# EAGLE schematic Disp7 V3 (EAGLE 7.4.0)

## Sheet 1 of 5: Powersupply
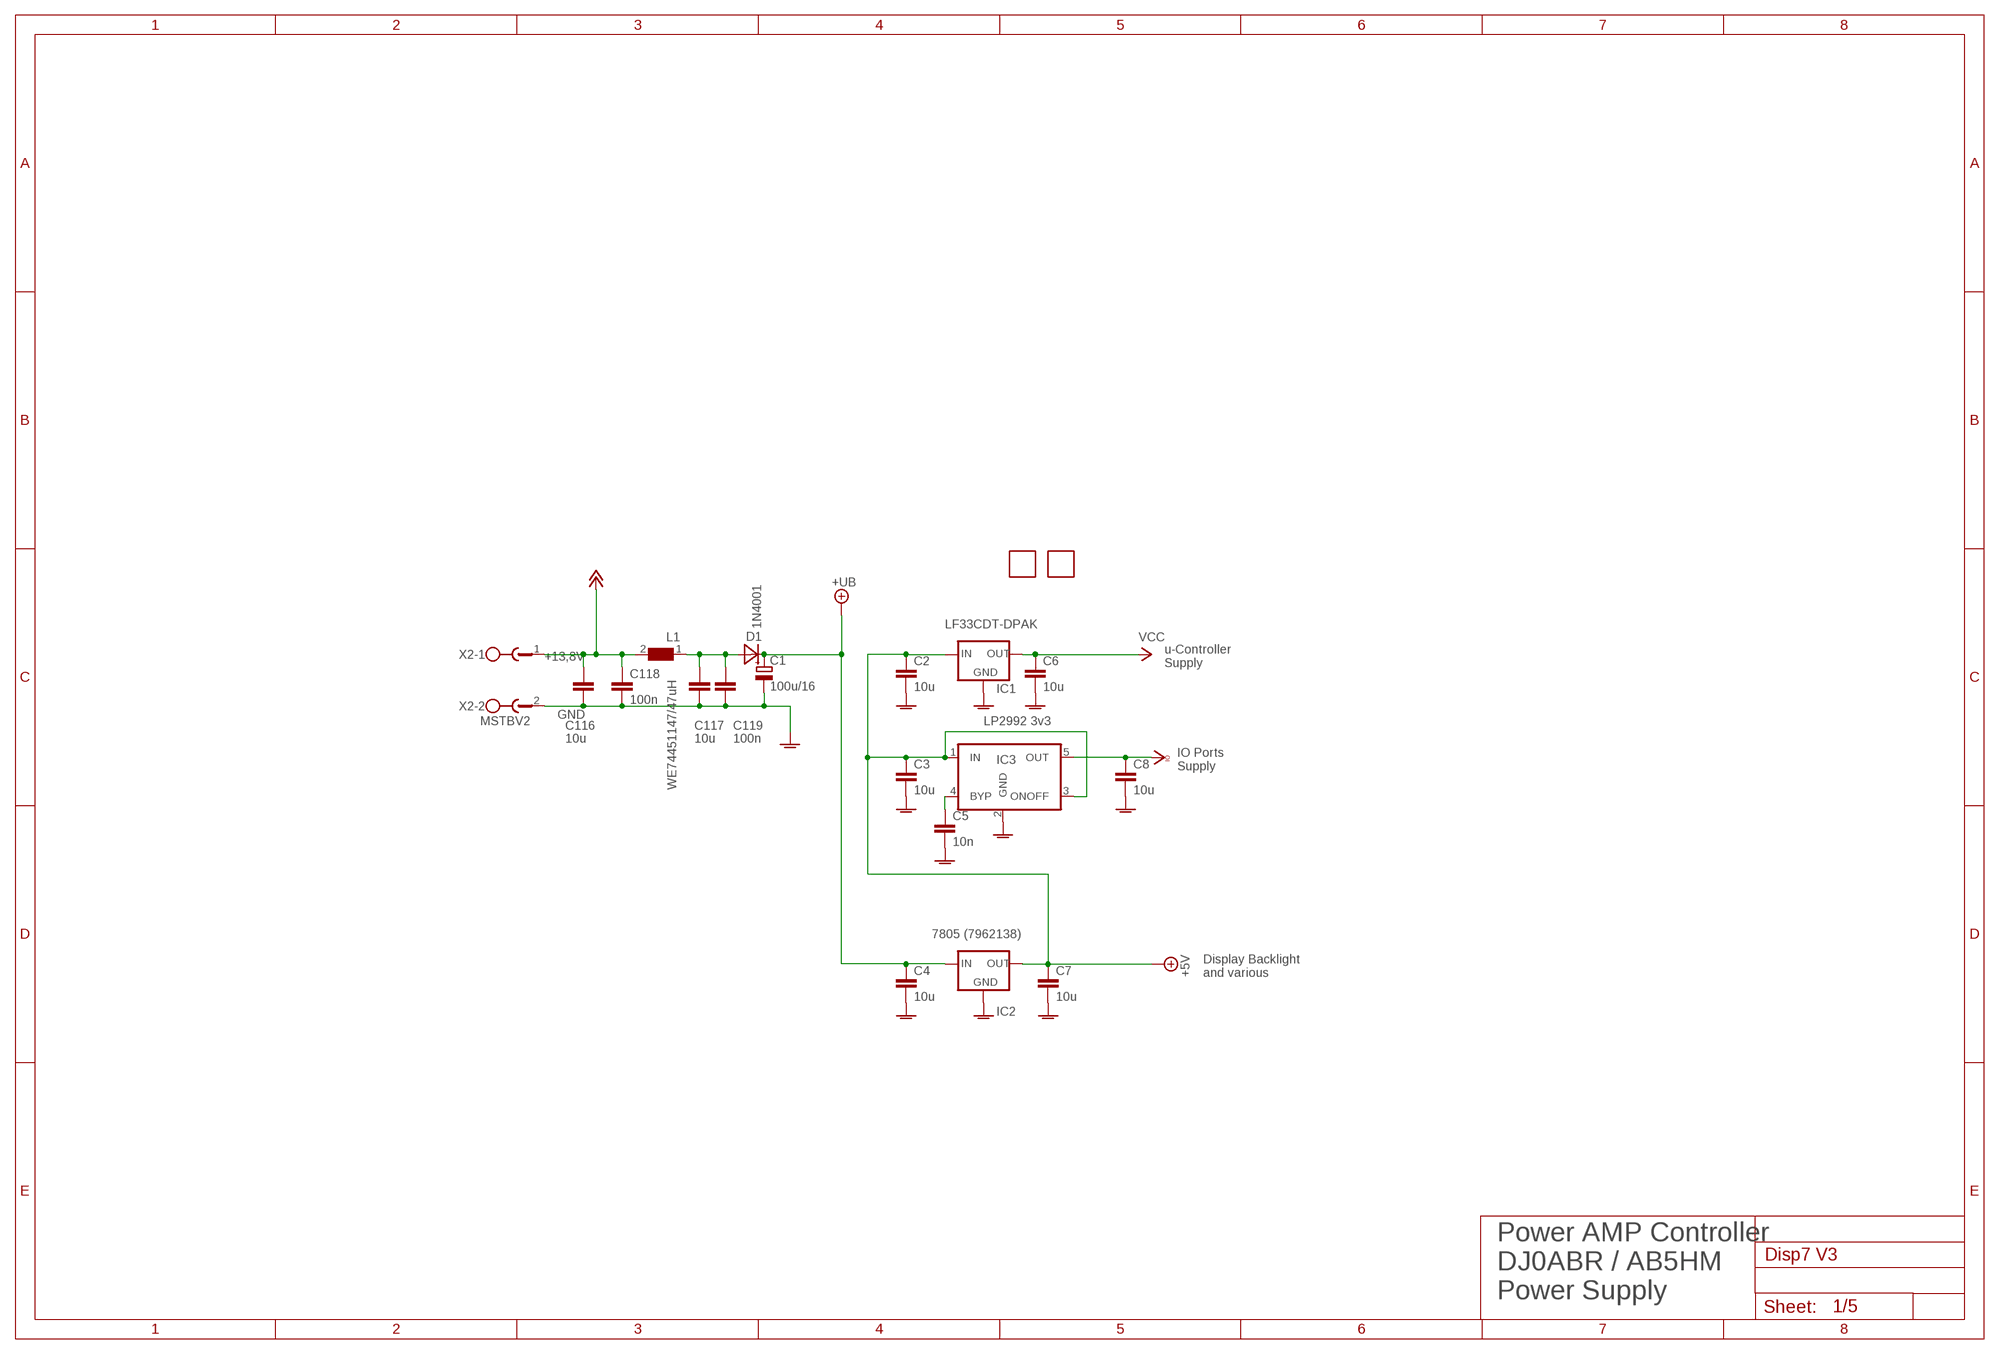
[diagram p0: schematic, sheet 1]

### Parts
C1  100u/16  CPOL-EUE2.5-7  [E2,5-7]
C2  10u  C-EUC0805  [C0805]
C3  10u  C-EUC0805  [C0805]
C4  10u  C-EUC0805  [C0805]
C5  10n  C-EUC0805  [C0805]
C6  10u  C-EUC0603  [C0603]
C7  10u  C-EUC0603  [C0603]
C8  10u  C-EUC0603  [C0603]
C116  10u  C-EUC0805  [C0805]
C117  10u  C-EUC0805  [C0805]
C118  100n  C-EUC0805  [C0805]
C119  100n  C-EUC0805  [C0805]
D1  1N4001  DIODE_GROSSSMD  [MELF]
FID1  FIDUCIAL  [FIDUCIAL]
FID2  FIDUCIAL  [FIDUCIAL]
IC1  LF33CDT-DPAK  LP2950CDT-5.0  [DPACK]
IC2  7805 (7962138)  78XXSWITCHREG  [78SR_SWITCHREG]
IC3  LP2992 3v3  UREG5  [SOT23-5]
L1  WE74451147/47uH  WE-PD3-74451147_S  [S]
X2  MSTBV2  [MSTBV2]

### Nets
+5V: C2.1 C3.1 C7.1 IC1.1(IN) IC2.3(OUT) IC3.1(IN) IC3.3(ONOFF) ; also sheet 3,4
+UB [Supply]: C1.+ C4.1 D1.1(C) IC2.1(IN) ; also sheet 3
AGND [AGND]: C1.- C2.2 C3.2 C4.2 C5.2 C6.2 C7.2 C8.2 C116.2 C117.2 C118.2 C119.2 IC1.4(GND) IC2.2(GND) IC3.2(GND) X2.2 ; supply symbol labelled  ; also sheet 2,3,4,5
N$47 [Supply]: C117.1 C119.1 D1.2(A) L1.1
N$125: C5.1 IC3.4(BYP)
PLUSZWOELF [Supply]: C116.1 C118.1 L1.2 X2.1 ; supply symbol labelled +12V ; also sheet 2
VCC [Supply]: C6.1 IC1.3(OUT) ; also sheet 2,4,5
VCCIO [Supply]: C8.1 IC3.5(OUT) ; supply symbol labelled  ; also sheet 3,4
Unconnected: FID1.P$1 FID2.P$1

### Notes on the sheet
- +13,8V
- u-Controller 
  Supply
- GND
- IO Ports
  Supply
- Display Backlight
  and various
- Power AMP Controller
  DJ0ABR / AB5HM
  Power Supply

## Sheet 2 of 5: IO Ports LED,PTT,Switch
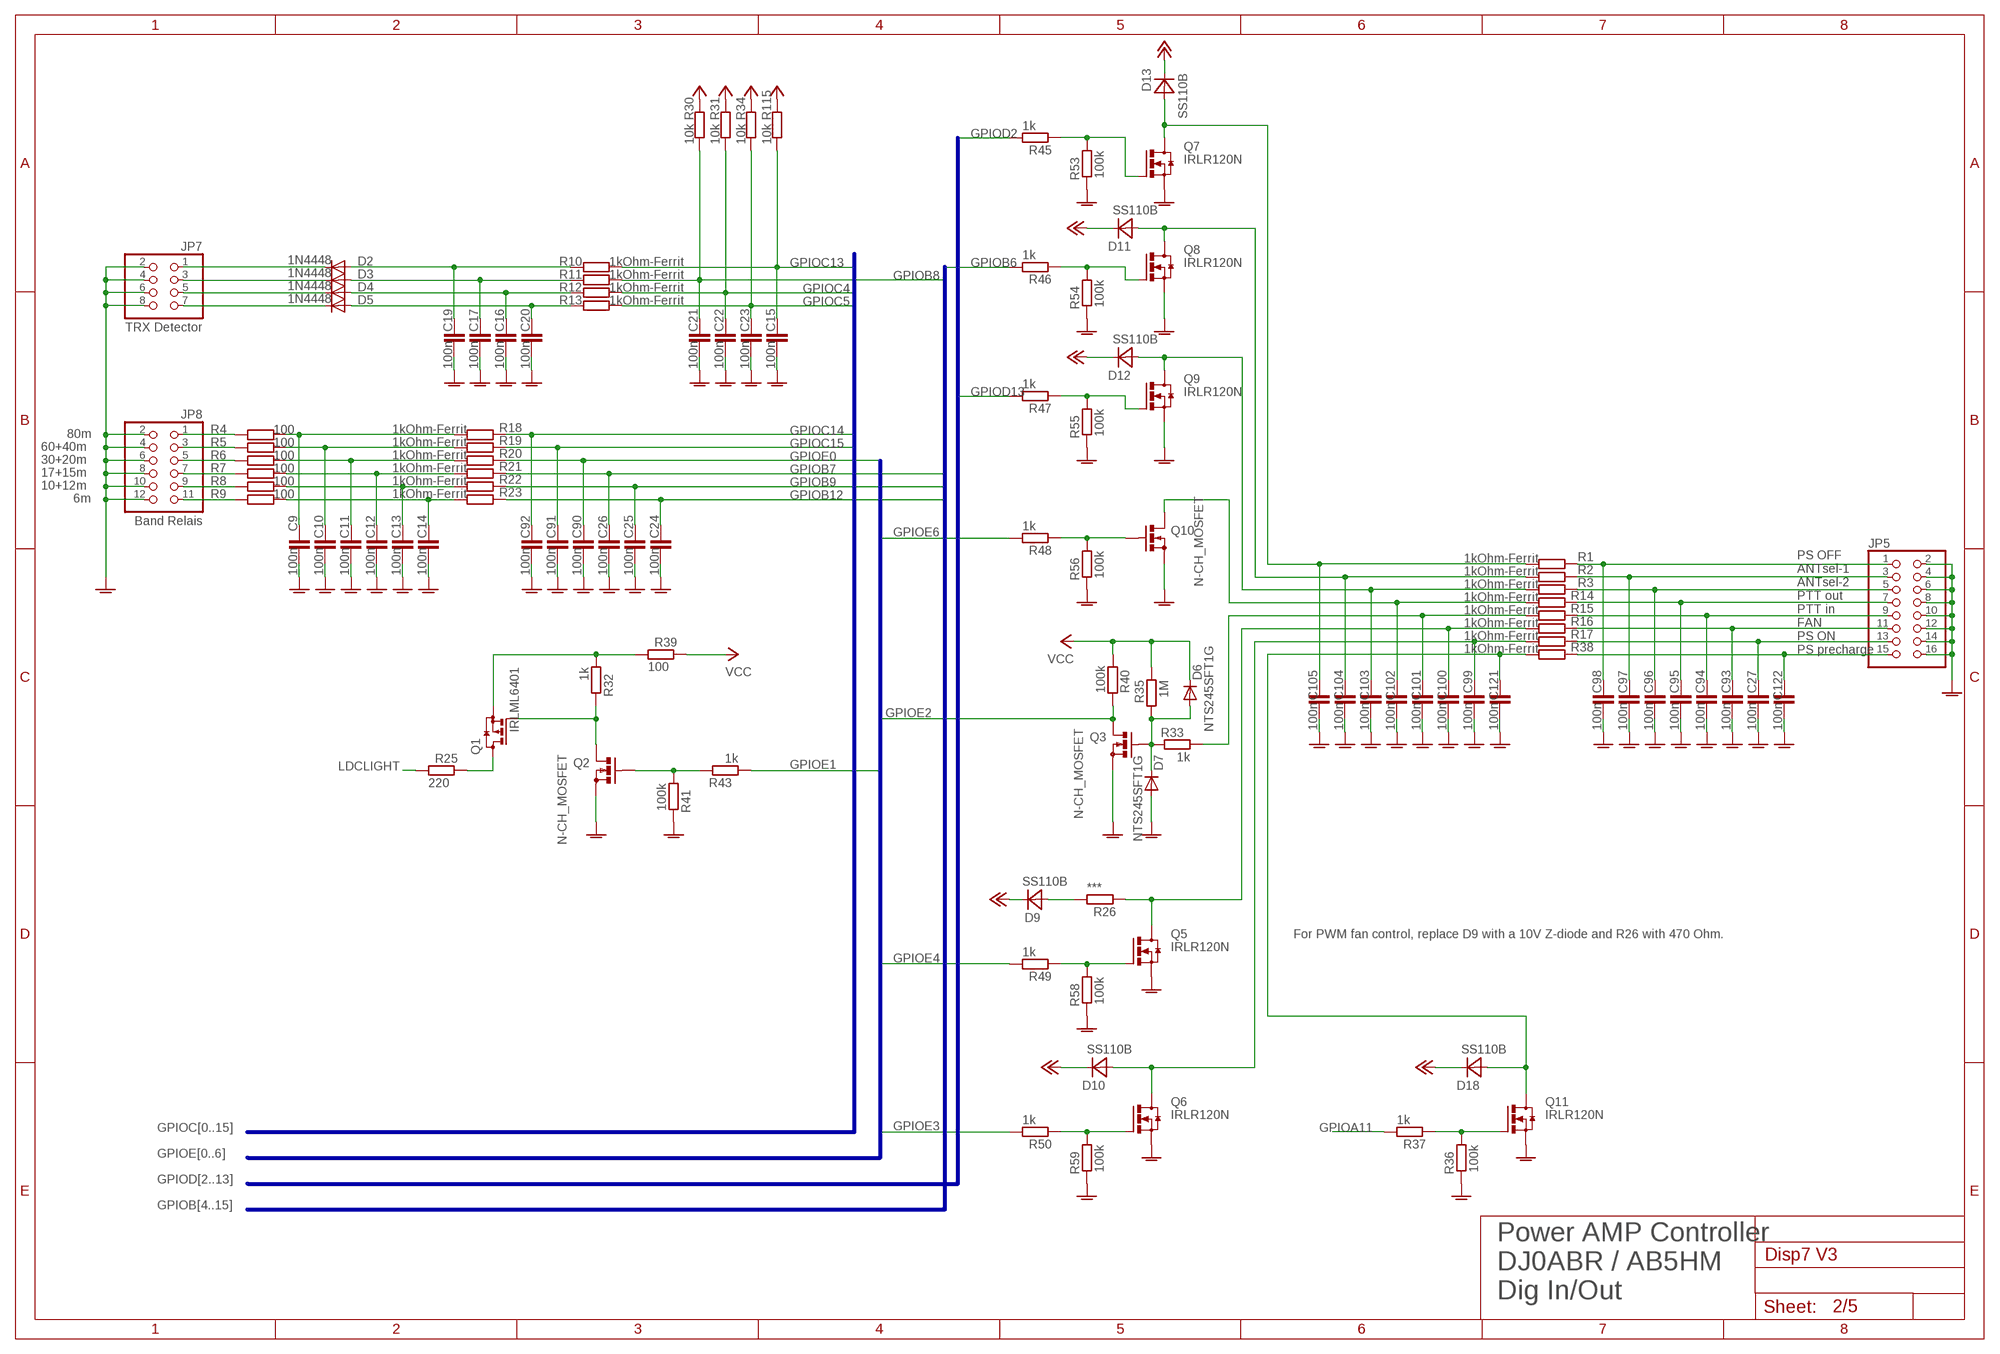
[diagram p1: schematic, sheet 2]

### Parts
C9  100n  C-EUC0805  [C0805]
C10  100n  C-EUC0805  [C0805]
C11  100n  C-EUC0805  [C0805]
C12  100n  C-EUC0805  [C0805]
C13  100n  C-EUC0805  [C0805]
C14  100n  C-EUC0805  [C0805]
C15  100n  C-EUC0805  [C0805]
C16  100n  C-EUC0805  [C0805]
C17  100n  C-EUC0805  [C0805]
C19  100n  C-EUC0805  [C0805]
C20  100n  C-EUC0805  [C0805]
C21  100n  C-EUC0805  [C0805]
C22  100n  C-EUC0805  [C0805]
C23  100n  C-EUC0805  [C0805]
C24  100n  C-EUC0805  [C0805]
C25  100n  C-EUC0805  [C0805]
C26  100n  C-EUC0805  [C0805]
C27  100n  C-EUC0805  [C0805]
C90  100n  C-EUC0805  [C0805]
C91  100n  C-EUC0805  [C0805]
C92  100n  C-EUC0805  [C0805]
C93  100n  C-EUC0805  [C0805]
C94  100n  C-EUC0805  [C0805]
C95  100n  C-EUC0805  [C0805]
C96  100n  C-EUC0805  [C0805]
C97  100n  C-EUC0805  [C0805]
C98  100n  C-EUC0805  [C0805]
C99  100n  C-EUC0805  [C0805]
C100  100n  C-EUC0805  [C0805]
C101  100n  C-EUC0805  [C0805]
C102  100n  C-EUC0805  [C0805]
C103  100n  C-EUC0805  [C0805]
C104  100n  C-EUC0805  [C0805]
C105  100n  C-EUC0805  [C0805]
C121  100n  C-EUC0805  [C0805]
C122  100n  C-EUC0805  [C0805]
D2  1N4448  DIODE-MINIMELF  [MINIMELF]
D3  1N4448  DIODE-MINIMELF  [MINIMELF]
D4  1N4448  DIODE-MINIMELF  [MINIMELF]
D5  1N4448  DIODE-MINIMELF  [MINIMELF]
D6  NTS245SFT1G  DIODE-MINIMELF  [MINIMELF]
D7  NTS245SFT1G  DIODE-MINIMELF  [MINIMELF]
D9  SS110B  DIODE_GROSSSMD  [MELF]
D10  SS110B  DIODE_GROSSSMD  [MELF]
D11  SS110B  DIODE_GROSSSMD  [MELF]
D12  SS110B  DIODE_GROSSSMD  [MELF]
D13  SS110B  DIODE_GROSSSMD  [MELF]
D18  SS110B  DIODE_GROSSSMD  [MELF]
JP5  PINHD-2X8/90  [2X08/90]
JP7  TRX Detector  PINHD-2X4/90  [2X04/90]
JP8  Band Relais  PINHD-2X6/90  [2X06/90]
Q1  IRLML6401  BSS84  [SOT23]
Q2  N-CH_MOSFET  BS170_SMD  [SOT23]
Q3  N-CH_MOSFET  BS170_SMD  [SOT23]
Q5  IRLR120N  [D-PAK_TO252AA]
Q6  IRLR120N  [D-PAK_TO252AA]
Q7  IRLR120N  [D-PAK_TO252AA]
Q8  IRLR120N  [D-PAK_TO252AA]
Q9  IRLR120N  [D-PAK_TO252AA]
Q10  N-CH_MOSFET  BS170_SMD  [SOT23]
Q11  IRLR120N  [D-PAK_TO252AA]
R1  1kOhm-Ferrit  R-EU_R0805  [R0805]
R2  1kOhm-Ferrit  R-EU_R0805  [R0805]
R3  1kOhm-Ferrit  R-EU_R0805  [R0805]
R4  100  R-EU_R0805  [R0805]
R5  100  R-EU_R0805  [R0805]
R6  100  R-EU_R0805  [R0805]
R7  100  R-EU_R0805  [R0805]
R8  100  R-EU_R0805  [R0805]
R9  100  R-EU_R0805  [R0805]
R10  1kOhm-Ferrit  R-EU_R0805  [R0805]
R11  1kOhm-Ferrit  R-EU_R0805  [R0805]
R12  1kOhm-Ferrit  R-EU_R0805  [R0805]
R13  1kOhm-Ferrit  R-EU_R0805  [R0805]
R14  1kOhm-Ferrit  R-EU_R0805  [R0805]
R15  1kOhm-Ferrit  R-EU_R0805  [R0805]
R16  1kOhm-Ferrit  R-EU_R0805  [R0805]
R17  1kOhm-Ferrit  R-EU_R0805  [R0805]
R18  1kOhm-Ferrit  R-EU_R0805  [R0805]
R19  1kOhm-Ferrit  R-EU_R0805  [R0805]
R20  1kOhm-Ferrit  R-EU_R0805  [R0805]
R21  1kOhm-Ferrit  R-EU_R0805  [R0805]
R22  1kOhm-Ferrit  R-EU_R0805  [R0805]
R23  1kOhm-Ferrit  R-EU_R0805  [R0805]
R25  220  R-EU_R0805  [R0805]
R26  ***  R-EU_R0805  [R0805]
R30  10k  R-EU_R0805  [R0805]
R31  10k  R-EU_R0805  [R0805]
R32  1k  R-EU_R0805  [R0805]
R33  1k  R-EU_R0805  [R0805]
R34  10k  R-EU_R0805  [R0805]
R35  1M  R-EU_R0805  [R0805]
R36  100k  R-EU_R0805  [R0805]
R37  1k  R-EU_R0805  [R0805]
R38  1kOhm-Ferrit  R-EU_R0805  [R0805]
R39  100  R-EU_R0805  [R0805]
R40  100k  R-EU_R0805  [R0805]
R41  100k  R-EU_R0805  [R0805]
R43  1k  R-EU_R0805  [R0805]
R45  1k  R-EU_R0805  [R0805]
R46  1k  R-EU_R0805  [R0805]
R47  1k  R-EU_R0805  [R0805]
R48  1k  R-EU_R0805  [R0805]
R49  1k  R-EU_R0805  [R0805]
R50  1k  R-EU_R0805  [R0805]
R53  100k  R-EU_R0805  [R0805]
R54  100k  R-EU_R0805  [R0805]
R55  100k  R-EU_R0805  [R0805]
R56  100k  R-EU_R0805  [R0805]
R58  100k  R-EU_R0805  [R0805]
R59  100k  R-EU_R0805  [R0805]
R115  10k  R-EU_R0805  [R0805]

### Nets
AGND [AGND]: C9.2 C10.2 C11.2 C12.2 C13.2 C14.2 C15.2 C16.2 C17.2 C19.2 C20.2 C21.2 C22.2 C23.2 C24.2 C25.2 C26.2 C27.2 C90.2 C91.2 C92.2 C93.2 C94.2 C95.2 C96.2 C97.2 C98.2 C99.2 C100.2 C101.2 C102.2 C103.2 C104.2 C105.2 C121.2 C122.2 D7.A JP5.2 JP5.4 JP5.6 JP5.8 JP5.10 JP5.12 JP5.14 JP5.16 JP7.2 JP7.4 JP7.6 JP7.8 JP8.2 JP8.4 JP8.6 JP8.8 JP8.10 JP8.12 Q2.2(S) Q3.2(S) Q5.3(S) Q6.3(S) Q7.3(S) Q8.3(S) Q9.3(S) Q10.2(S) Q11.3(S) R36.2 R41.2 R53.2 R54.2 R55.2 R56.2 R58.2 R59.2 ; supply symbol labelled  ; also sheet 1,3,4,5
GPIOA11: R37.1 ; also sheet 4
GPIOB6: R46.1 ; also sheet 4
GPIOB7: C26.1 R21.1 ; also sheet 4
GPIOB8: C21.1 R11.2 R30.1 ; also sheet 4
GPIOB9: C25.1 R22.1 ; also sheet 4
GPIOB12: C24.1 R23.1 ; also sheet 4
GPIOC4: C22.1 R12.2 R31.1 ; also sheet 4
GPIOC5: C23.1 R13.2 R34.1 ; also sheet 4
GPIOC13: C15.1 R10.2 R115.1 ; also sheet 4
GPIOC14: C92.1 R18.1 ; also sheet 4
GPIOC15: C91.1 R19.1 ; also sheet 4
GPIOD2: R45.1 ; also sheet 4
GPIOD13: R47.1 ; also sheet 4
GPIOE0: C90.1 R20.1 ; also sheet 4
GPIOE1: R43.1 ; also sheet 4
GPIOE2: Q3.3(D) R40.1 ; also sheet 4
GPIOE3: R50.1 ; also sheet 4
GPIOE4: R49.1 ; also sheet 4
GPIOE6: R48.1 ; also sheet 4
LDCLIGHT: R25.1 ; also sheet 4
N$1: Q10.1(G) R48.2 R56.1
N$2: C102.1 Q10.3(D) R14.2
N$4: D6.A D7.C Q3.1(G) R33.2 R35.2
N$6: Q2.1(G) R41.1 R43.2
N$8: Q1.1(G) Q2.3(D) R32.2
N$10: Q1.3(D) R25.2
N$12: JP8.1 R4.1
N$14: C121.1 D18.2(A) Q11.4(D) R38.2
N$27: Q11.1(G) R36.1 R37.2
N$29: C122.1 JP5.15 R38.1
N$33: C98.1 JP5.1 R1.1
N$45: Q9.1(G) R47.2 R55.1
N$46: C103.1 D12.2(A) Q9.4(D) R3.2
N$50: C97.1 JP5.3 R2.1
N$51: C96.1 JP5.5 R3.1
N$52: C95.1 JP5.7 R14.1
N$56: C94.1 JP5.9 R15.1
N$57: C93.1 JP5.11 R16.1
N$58: D3.C JP7.3
N$59: D4.C JP7.5
N$60: D5.C JP7.7
N$63: C27.1 JP5.13 R17.1
N$65: D9.2(A) R26.1
N$90: C9.1 R4.2 R18.2
N$94: C14.1 R9.2 R23.2
N$95: C13.1 R8.2 R22.2
N$98: C12.1 R7.2 R21.2
N$99: C11.1 R6.2 R20.2
N$100: C10.1 R5.2 R19.2
N$105: Q1.2(S) R32.1 R39.1
N$106: D2.C JP7.1
N$109: Q8.1(G) R46.2 R54.1
N$110: C104.1 D11.2(A) Q8.4(D) R2.2
N$115: JP8.3 R5.1
N$116: JP8.5 R6.1
N$118: Q7.1(G) R45.2 R53.1
N$119: JP8.7 R7.1
N$120: JP8.9 R8.1
N$121: JP8.11 R9.1
N$122: C105.1 D13.2(A) Q7.4(D) R1.2
N$126: C19.1 D2.A R10.1
N$127: C17.1 D3.A R11.1
N$128: C16.1 D4.A R12.1
N$129: C20.1 D5.A R13.1
N$132: C100.1 Q5.4(D) R16.2 R26.2
N$134: Q5.1(G) R49.2 R58.1
N$135: C99.1 D10.2(A) Q6.4(D) R17.2
N$136: Q6.1(G) R50.2 R59.1
PLUSZWOELF [Supply]: D9.1(C) D10.1(C) D11.1(C) D12.1(C) D13.1(C) D18.1(C) ; supply symbol labelled +12V ; also sheet 1
PTT: C101.1 R15.2 R33.1
VCC [Supply]: D6.C R30.2 R31.2 R34.2 R35.1 R39.2 R40.2 R115.2 ; also sheet 1,4,5

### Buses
GPIOC[0..15]
GPIOE[0..6]
GPIOD[2..13]
GPIOB[4..15]

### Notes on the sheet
- 80m
- 60+40m
- 30+20m
- 17+15m
- 10+12m
- 6m
- PS OFF
  ANTsel-1
  ANTsel-2
  PTT out
  PTT in
  FAN
  PS ON
  PS precharge
- For PWM fan control, replace D9 with a 10V Z-diode and R26 with 470 Ohm.
- Power AMP Controller
  DJ0ABR / AB5HM
  Dig In/Out

## Sheet 3 of 5: ANALOG
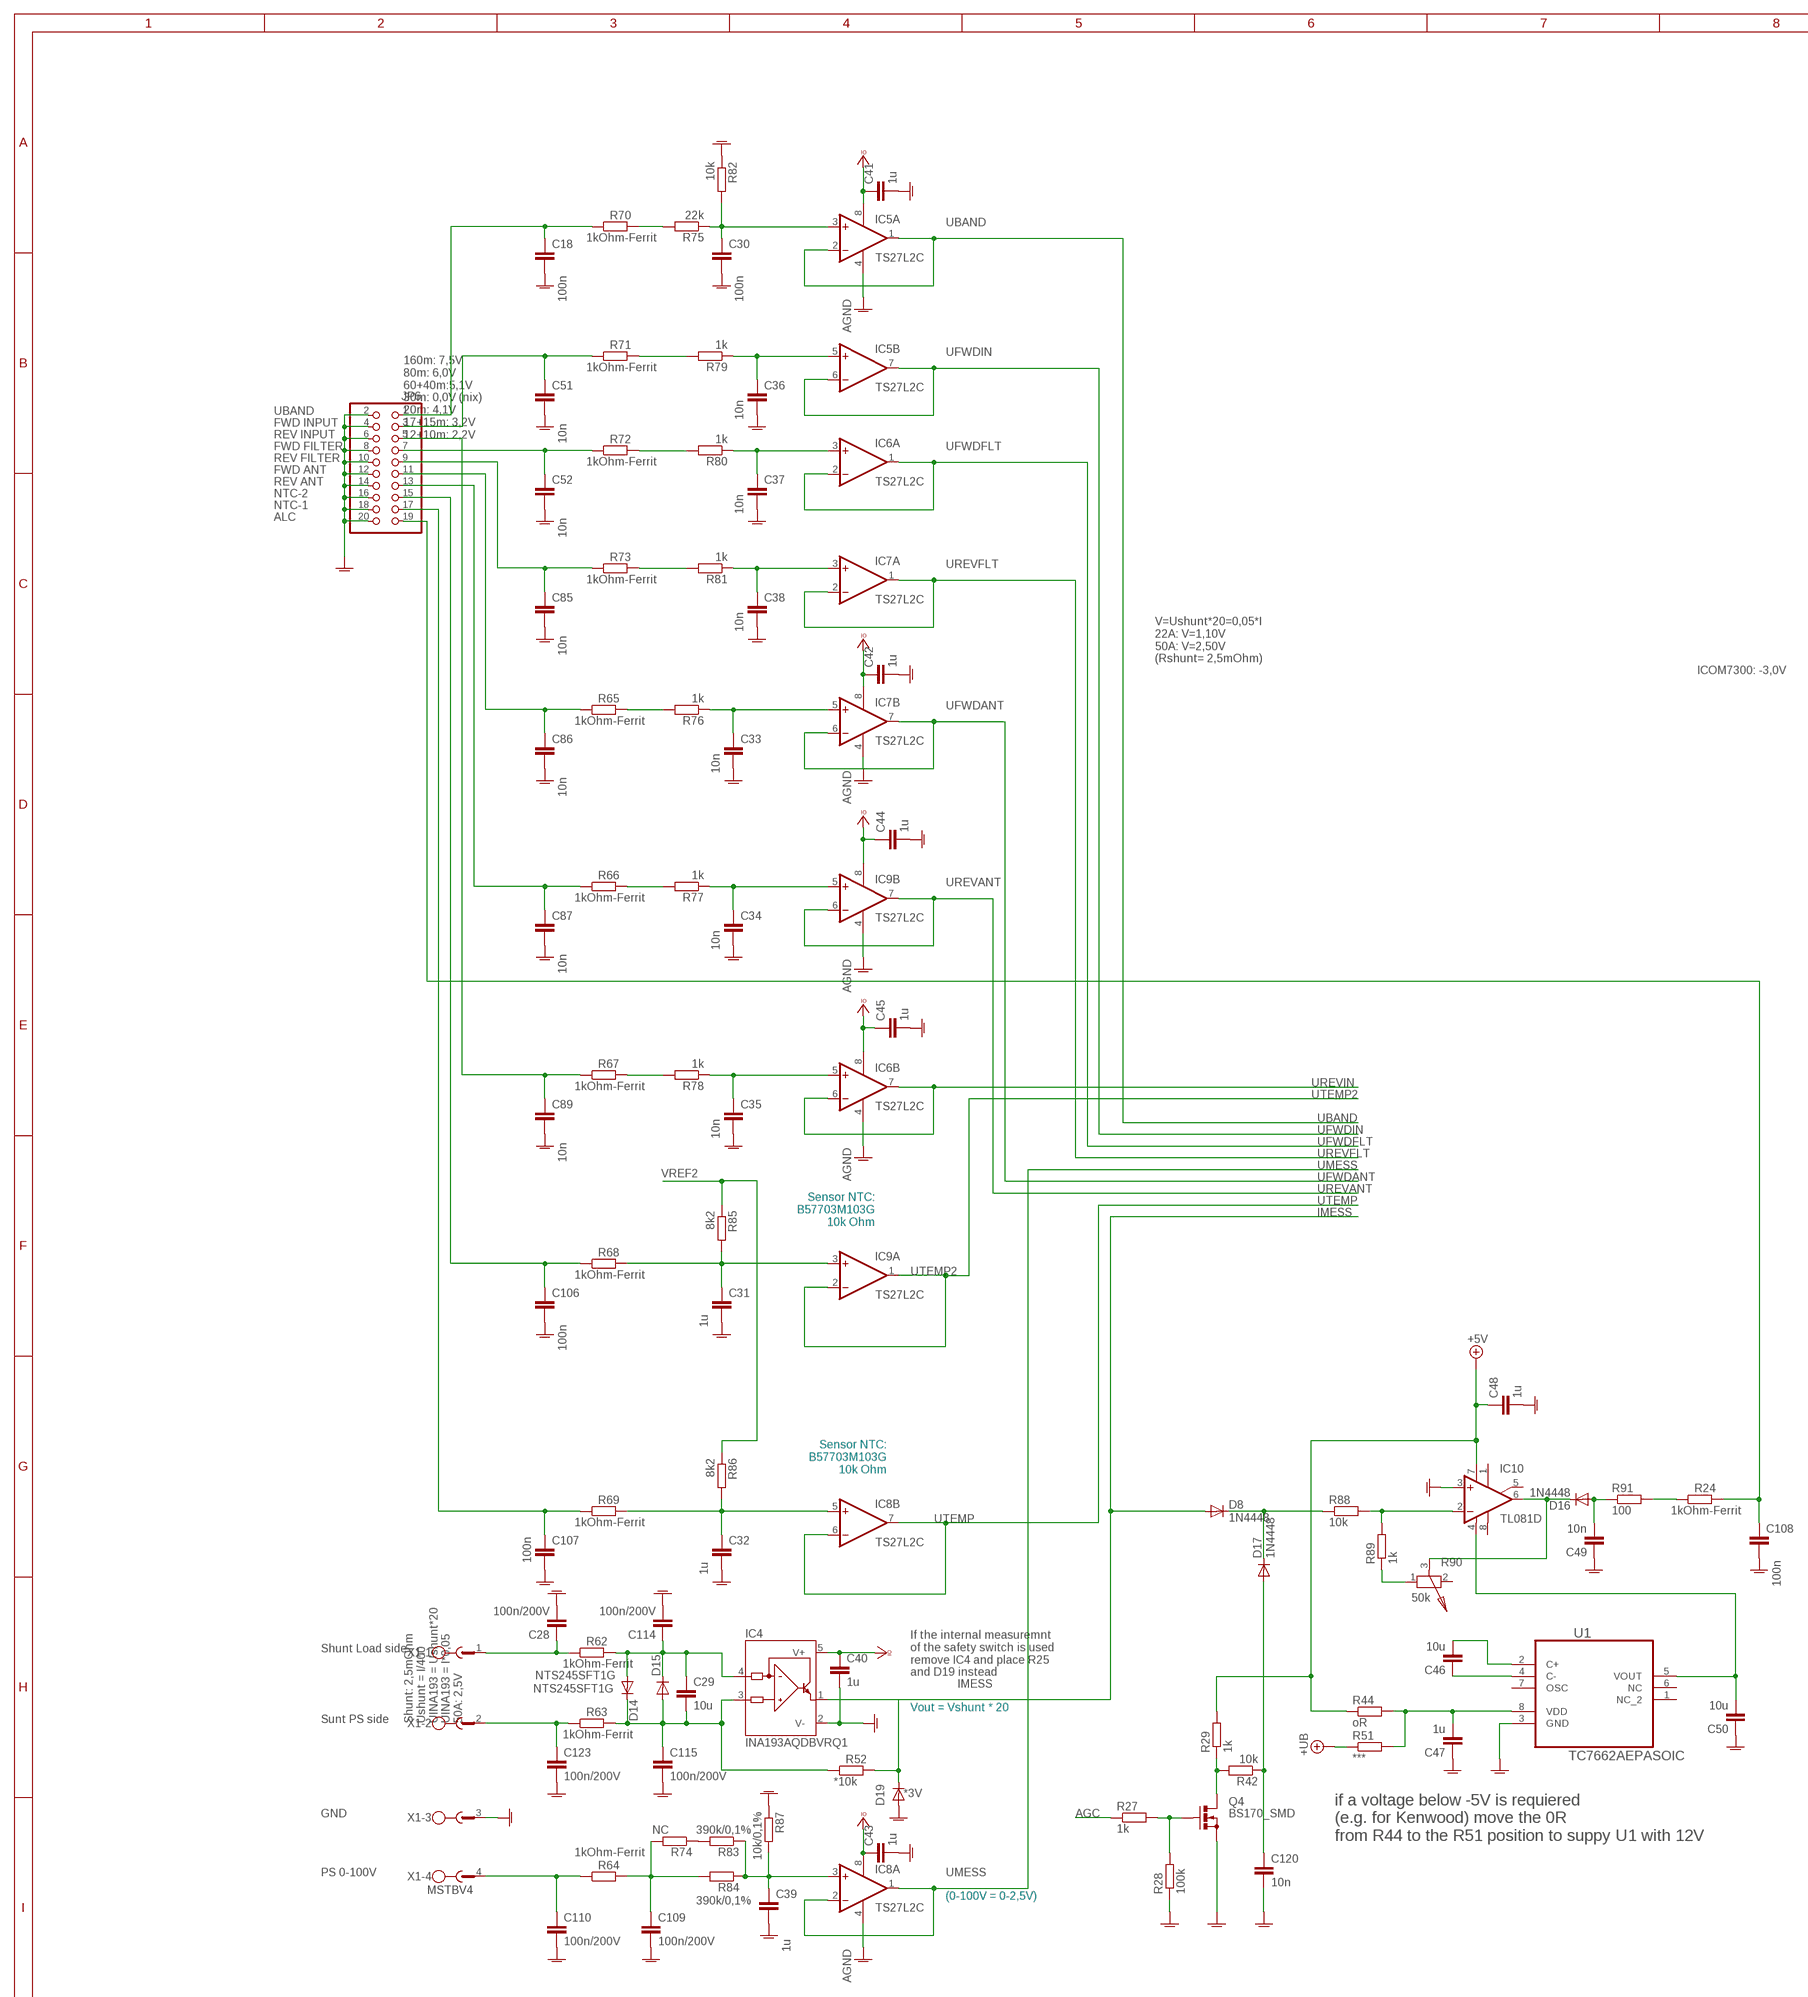
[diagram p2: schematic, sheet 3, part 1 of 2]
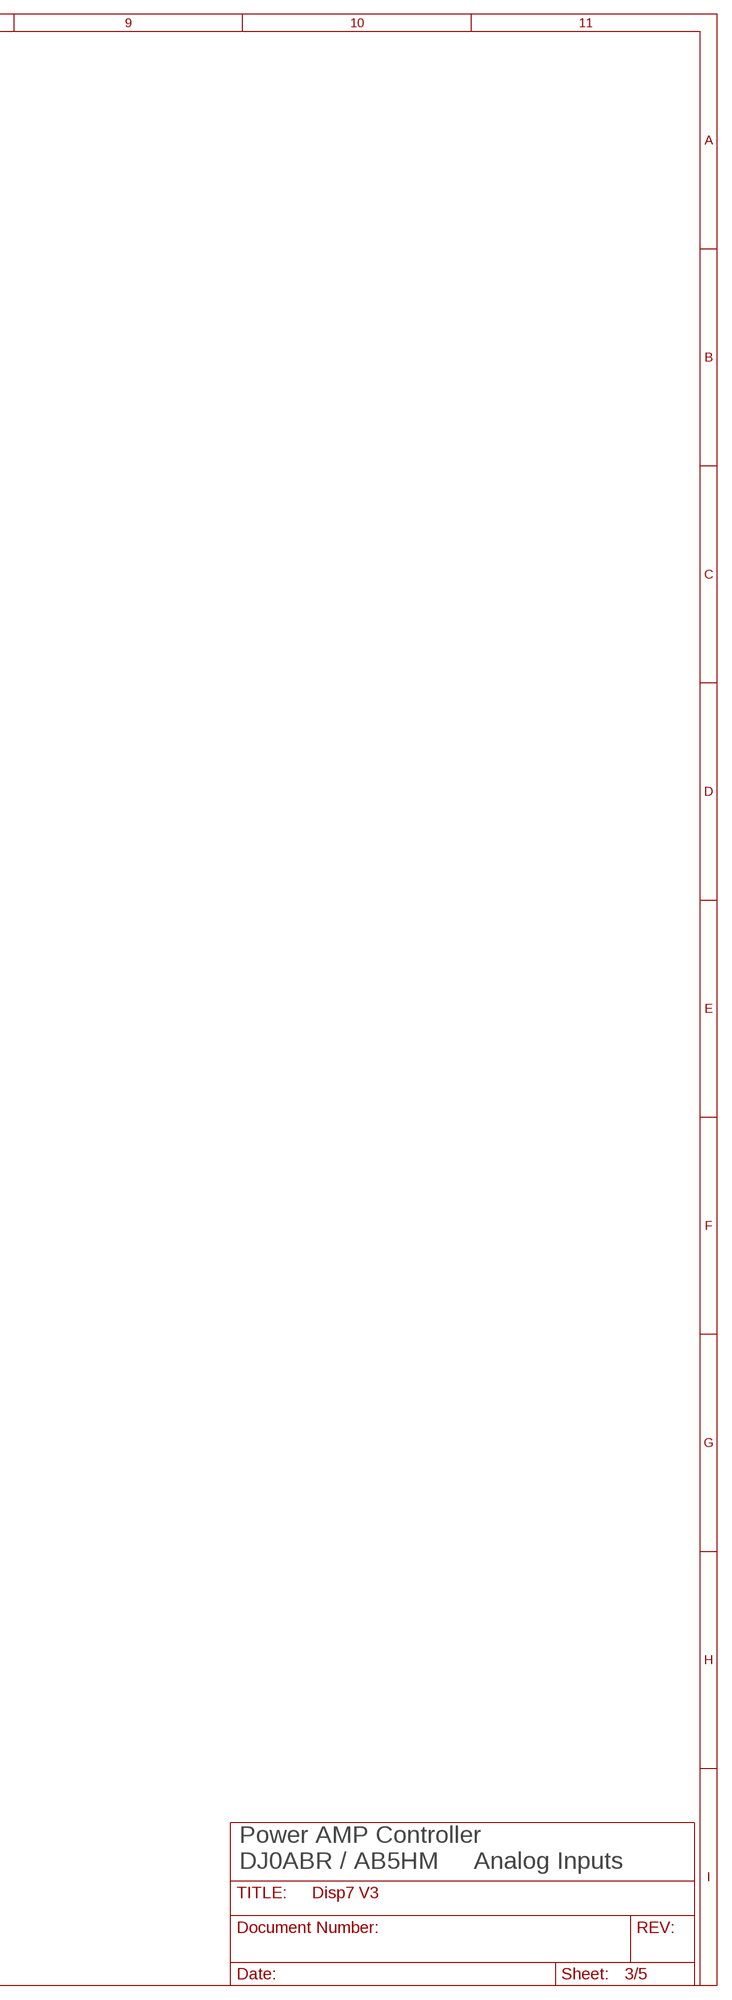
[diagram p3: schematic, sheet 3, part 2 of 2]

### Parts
C18  100n  C-EUC0805  [C0805]
C28  100n/200V  C-EUC1206  [C1206]
C29  10u  C-EUC0805  [C0805]
C30  100n  C-EUC0805  [C0805]
C31  1u  C-EUC0805  [C0805]
C32  1u  C-EUC0805  [C0805]
C33  10n  C-EUC0805  [C0805]
C34  10n  C-EUC0805  [C0805]
C35  10n  C-EUC0805  [C0805]
C36  10n  C-EUC0805  [C0805]
C37  10n  C-EUC0805  [C0805]
C38  10n  C-EUC0805  [C0805]
C39  1u  C-EUC0805  [C0805]
C40  1u  C-EUC0805  [C0805]
C41  1u  C-EUC0805  [C0805]
C42  1u  C-EUC0805  [C0805]
C43  1u  C-EUC0805  [C0805]
C44  1u  C-EUC0805  [C0805]
C45  1u  C-EUC0805  [C0805]
C46  10u  C-EUC0805  [C0805]
C47  1u  C-EUC0805  [C0805]
C48  1u  C-EUC0805  [C0805]
C49  10n  C-EUC0805  [C0805]
C50  10u  C-EUC0805  [C0805]
C51  10n  C-EUC0805  [C0805]
C52  10n  C-EUC0805  [C0805]
C85  10n  C-EUC0805  [C0805]
C86  10n  C-EUC0805  [C0805]
C87  10n  C-EUC0805  [C0805]
C89  10n  C-EUC0805  [C0805]
C106  100n  C-EUC0805  [C0805]
C107  100n  C-EUC0805  [C0805]
C108  100n  C-EUC0805  [C0805]
C109  100n/200V  C-EUC1206  [C1206]
C110  100n/200V  C-EUC1206  [C1206]
C114  100n/200V  C-EUC1206  [C1206]
C115  100n/200V  C-EUC1206  [C1206]
C120  10n  C-EUC0805  [C0805]
C123  100n/200V  C-EUC1206  [C1206]
D8  1N4448  DIODE-MINIMELF  [MINIMELF]
D14  NTS245SFT1G  DIODE-MINIMELF  [MINIMELF]
D15  NTS245SFT1G  DIODE-MINIMELF  [MINIMELF]
D16  1N4448  DIODE-MINIMELF  [MINIMELF]
D17  1N4448  DIODE-MINIMELF  [MINIMELF]
D19  *3V  DIODE-MINIMELF  [MINIMELF]
IC4  INA193AQDBVRQ1  INA168  [SOT23-5]
IC5  TS27L2C  LM358D  [SO08]
IC6  TS27L2C  LM358D  [SO08]
IC7  TS27L2C  LM358D  [SO08]
IC8  TS27L2C  LM358D  [SO08]
IC9  TS27L2C  LM358D  [SO08]
IC10  TL081D  [SO08]
JP6  PINHD-2X10/90  [2X10/90]
Q4  BS170_SMD  [SOT23]
R24  1kOhm-Ferrit  R-EU_R0805  [R0805]
R27  1k  R-EU_R0805  [R0805]
R28  100k  R-EU_R0805  [R0805]
R29  1k  R-EU_R0805  [R0805]
R42  10k  R-EU_R0805  [R0805]
R44  oR  R-EU_R0805  [R0805]
R51  ***  R-EU_R0805  [R0805]
R52  *10k  R-EU_R0805  [R0805]
R62  1kOhm-Ferrit  R-EU_R0805  [R0805]
R63  1kOhm-Ferrit  R-EU_R0805  [R0805]
R64  1kOhm-Ferrit  R-EU_R0805  [R0805]
R65  1kOhm-Ferrit  R-EU_R0805  [R0805]
R66  1kOhm-Ferrit  R-EU_R0805  [R0805]
R67  1kOhm-Ferrit  R-EU_R0805  [R0805]
R68  1kOhm-Ferrit  R-EU_R0805  [R0805]
R69  1kOhm-Ferrit  R-EU_R0805  [R0805]
R70  1kOhm-Ferrit  R-EU_R0805  [R0805]
R71  1kOhm-Ferrit  R-EU_R0805  [R0805]
R72  1kOhm-Ferrit  R-EU_R0805  [R0805]
R73  1kOhm-Ferrit  R-EU_R0805  [R0805]
R74  NC  R-EU_R0805  [R0805]
R75  22k  R-EU_R0805  [R0805]
R76  1k  R-EU_R0805  [R0805]
R77  1k  R-EU_R0805  [R0805]
R78  1k  R-EU_R0805  [R0805]
R79  1k  R-EU_R0805  [R0805]
R80  1k  R-EU_R0805  [R0805]
R81  1k  R-EU_R0805  [R0805]
R82  10k  R-EU_R0805  [R0805]
R83  390k/0,1%  R-EU_R0805  [R0805]
R84  390k/0,1%  R-EU_R0805  [R0805]
R85  8k2  R-EU_R0805  [R0805]
R86  8k2  R-EU_R0805  [R0805]
R87  10k/0,1%  R-EU_R0805  [R0805]
R88  10k  R-EU_R0805  [R0805]
R89  1k  R-EU_R0805  [R0805]
R90  50k  MINIPOTI-S  [MINIPOTI]
R91  100  R-EU_R0805  [R0805]
U1  TC7662AEPASOIC  [SO-8]
X1  MSTBV4  [MSTBV4]

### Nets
+5V: C48.1 IC10.7(V+) R29.2 R44.1 ; also sheet 1,4
+UB [Supply]: R51.1 ; also sheet 1
AGC: R27.1 ; also sheet 4
AGND [AGND]: C18.2 C28.2 C30.2 C31.2 C32.2 C33.2 C34.2 C35.2 C36.2 C37.2 C38.2 C39.2 C40.2 C41.2 C42.2 C43.2 C44.2 C45.2 C47.1 C48.2 C49.1 C50.1 C51.2 C52.2 C85.2 C86.2 C87.2 C89.2 C106.2 C107.2 C108.2 C109.2 C110.2 C114.2 C115.2 C120.2 C123.2 D19.A IC4.2(V-) IC5.4(P:V-) IC6.4(P:V-) IC7.4(P:V-) IC8.4(P:V-) IC9.4(P:V-) IC10.3(+IN) JP6.2 JP6.4 JP6.6 JP6.8 JP6.10 JP6.12 JP6.14 JP6.16 JP6.18 JP6.20 Q4.2(S) R28.1 R82.1 R87.1 U1.3(GND) ; supply symbol labelled  ; also sheet 1,2,4,5
IMESS: D8.A D19.C IC4.1(OUT) R52.2 ; also sheet 4
N$3: R24.1 R91.2
N$5: D8.C D17.C R88.1
N$7: Q4.1(G) R27.2 R28.2
N$11: C120.1 D17.A R42.1
N$19: R70.2 R75.2
N$21: R71.2 R79.2
N$38: R72.2 R80.2
N$44: Q4.3(D) R29.1 R42.2
N$49: C30.1 IC5.3(A:+IN) R75.1 R82.2
N$53: C18.1 JP6.1 R70.1
N$54: R73.2 R81.2
N$55: C109.1 R64.2 R74.2 R84.2
N$61: R65.2 R76.2
N$62: R66.2 R77.2
N$64: C39.1 IC8.3(A:+IN) R83.1 R84.1 R87.2
N$66: C47.2 R44.2 R51.2 U1.8(VDD)
N$67: C123.1 R63.1 X1.2
N$72: C33.1 IC7.5(B:+IN) R76.1
N$73: C86.1 JP6.11 R65.1
N$75: C34.1 IC9.5(B:+IN) R77.1
N$76: C87.1 JP6.13 R66.1
N$78: C29.1 C114.1 D14.A D15.C IC4.4(IN-) R62.2
N$79: C29.2 C115.1 D14.C D15.A IC4.3(IN+) R52.1 R63.2
N$80: C28.1 R62.1 X1.1
N$81: C110.1 R64.1 X1.4
N$82: C32.1 IC8.5(B:+IN) R69.2 R86.2
N$83: C107.1 JP6.17 R69.1
N$85: C38.1 IC7.3(A:+IN) R81.1
N$86: C85.1 JP6.9 R73.1
N$88: C37.1 IC6.3(A:+IN) R80.1
N$89: C52.1 JP6.7 R72.1
N$91: C36.1 IC5.5(B:+IN) R79.1
N$92: C51.1 JP6.3 R71.1
N$108: C35.1 IC6.5(B:+IN) R78.1
N$111: C89.1 JP6.5 R67.1
N$112: R67.2 R78.2
N$113: C31.1 IC9.3(A:+IN) R68.2 R85.2
N$114: C106.1 JP6.15 R68.1
N$124: R74.1 R83.2
N$144: C46.1 U1.4(C-)
N$145: C46.2 U1.2(C+)
N$146: C50.2 IC10.4(V-) U1.5(VOUT)
N$147: D16.C IC10.6(OUT) R90.3
N$148: C108.1 JP6.19 R24.2
N$149: IC10.2(-IN) R88.2 R89.2
N$150: R89.1 R90.1
N$151: C49.2 D16.A R91.1
UBAND: IC5.1(A:OUT) IC5.2(A:-IN) ; also sheet 4
UFWDANT: IC7.6(B:-IN) IC7.7(B:OUT) ; also sheet 4
UFWDFLT: IC6.1(A:OUT) IC6.2(A:-IN) ; also sheet 4
UFWDIN: IC5.6(B:-IN) IC5.7(B:OUT) ; also sheet 4
UMESS: IC8.1(A:OUT) IC8.2(A:-IN) ; also sheet 4
UREVANT: IC9.6(B:-IN) IC9.7(B:OUT) ; also sheet 4
UREVFLT: IC7.1(A:OUT) IC7.2(A:-IN) ; also sheet 4
UREVIN: IC6.6(B:-IN) IC6.7(B:OUT) ; also sheet 4
UTEMP: IC8.6(B:-IN) IC8.7(B:OUT) ; also sheet 4
UTEMP2: IC9.1(A:OUT) IC9.2(A:-IN) ; also sheet 4
VCCIO [Supply]: C40.1 C41.1 C42.1 C43.1 C44.1 C45.1 IC4.5(V+) IC5.8(P:V+) IC6.8(P:V+) IC7.8(P:V+) IC8.8(P:V+) IC9.8(P:V+) ; supply symbol labelled  ; also sheet 1,4
VREF2: R85.1 R86.1 ; also sheet 4
Unconnected: IC10.1(ON1) IC10.5(ON2) IC10.8(OPT) R90.2 U1.1(NC_2) U1.6(NC) U1.7(OSC) X1.3

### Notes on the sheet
- UBAND
- FWD INPUT
- REV INPUT
- 160m: 7,5V
  80m: 6,0V
  60+40m:5,1V
  30m: 0,0V (nix)
  20m: 4,1V
  17+15m: 3,2V
  12+10m: 2,2V
- FWD FILTER
- REV FILTER
- FWD ANT
- REV ANT
- NTC-2
- NTC-1
- ALC
- V=Ushunt*20=0,05*I
  22A: V=1,10V
  50A: V=2,50V
  (Rshunt= 2,5mOhm)
- ICOM7300: -3,0V
- Sensor NTC:
  B57703M103G
  10k Ohm
- Sensor NTC:
  B57703M103G
  10k Ohm
- Shunt Load side
- If the internal measuremnt
  of the safety switch is used
  remove IC4 and place R25 
  and D19 instead
- Vout = Vshunt * 20
- Sunt PS side
- Shunt: 2,5mOhm
  Ushunt = I/400
  UINA193 = Ushunt*20
  UINA193 = I*0,05
  50A: 2,5V
- GND
- if a voltage below -5V is requiered
  (e.g. for Kenwood) move the 0R 
  from R44 to the R51 position to suppy U1 with 12V
- PS 0-100V
- (0-100V = 0-2,5V)
- Power AMP Controller
  DJ0ABR / AB5HM     Analog Inputs

## Sheet 4 of 5: CPU
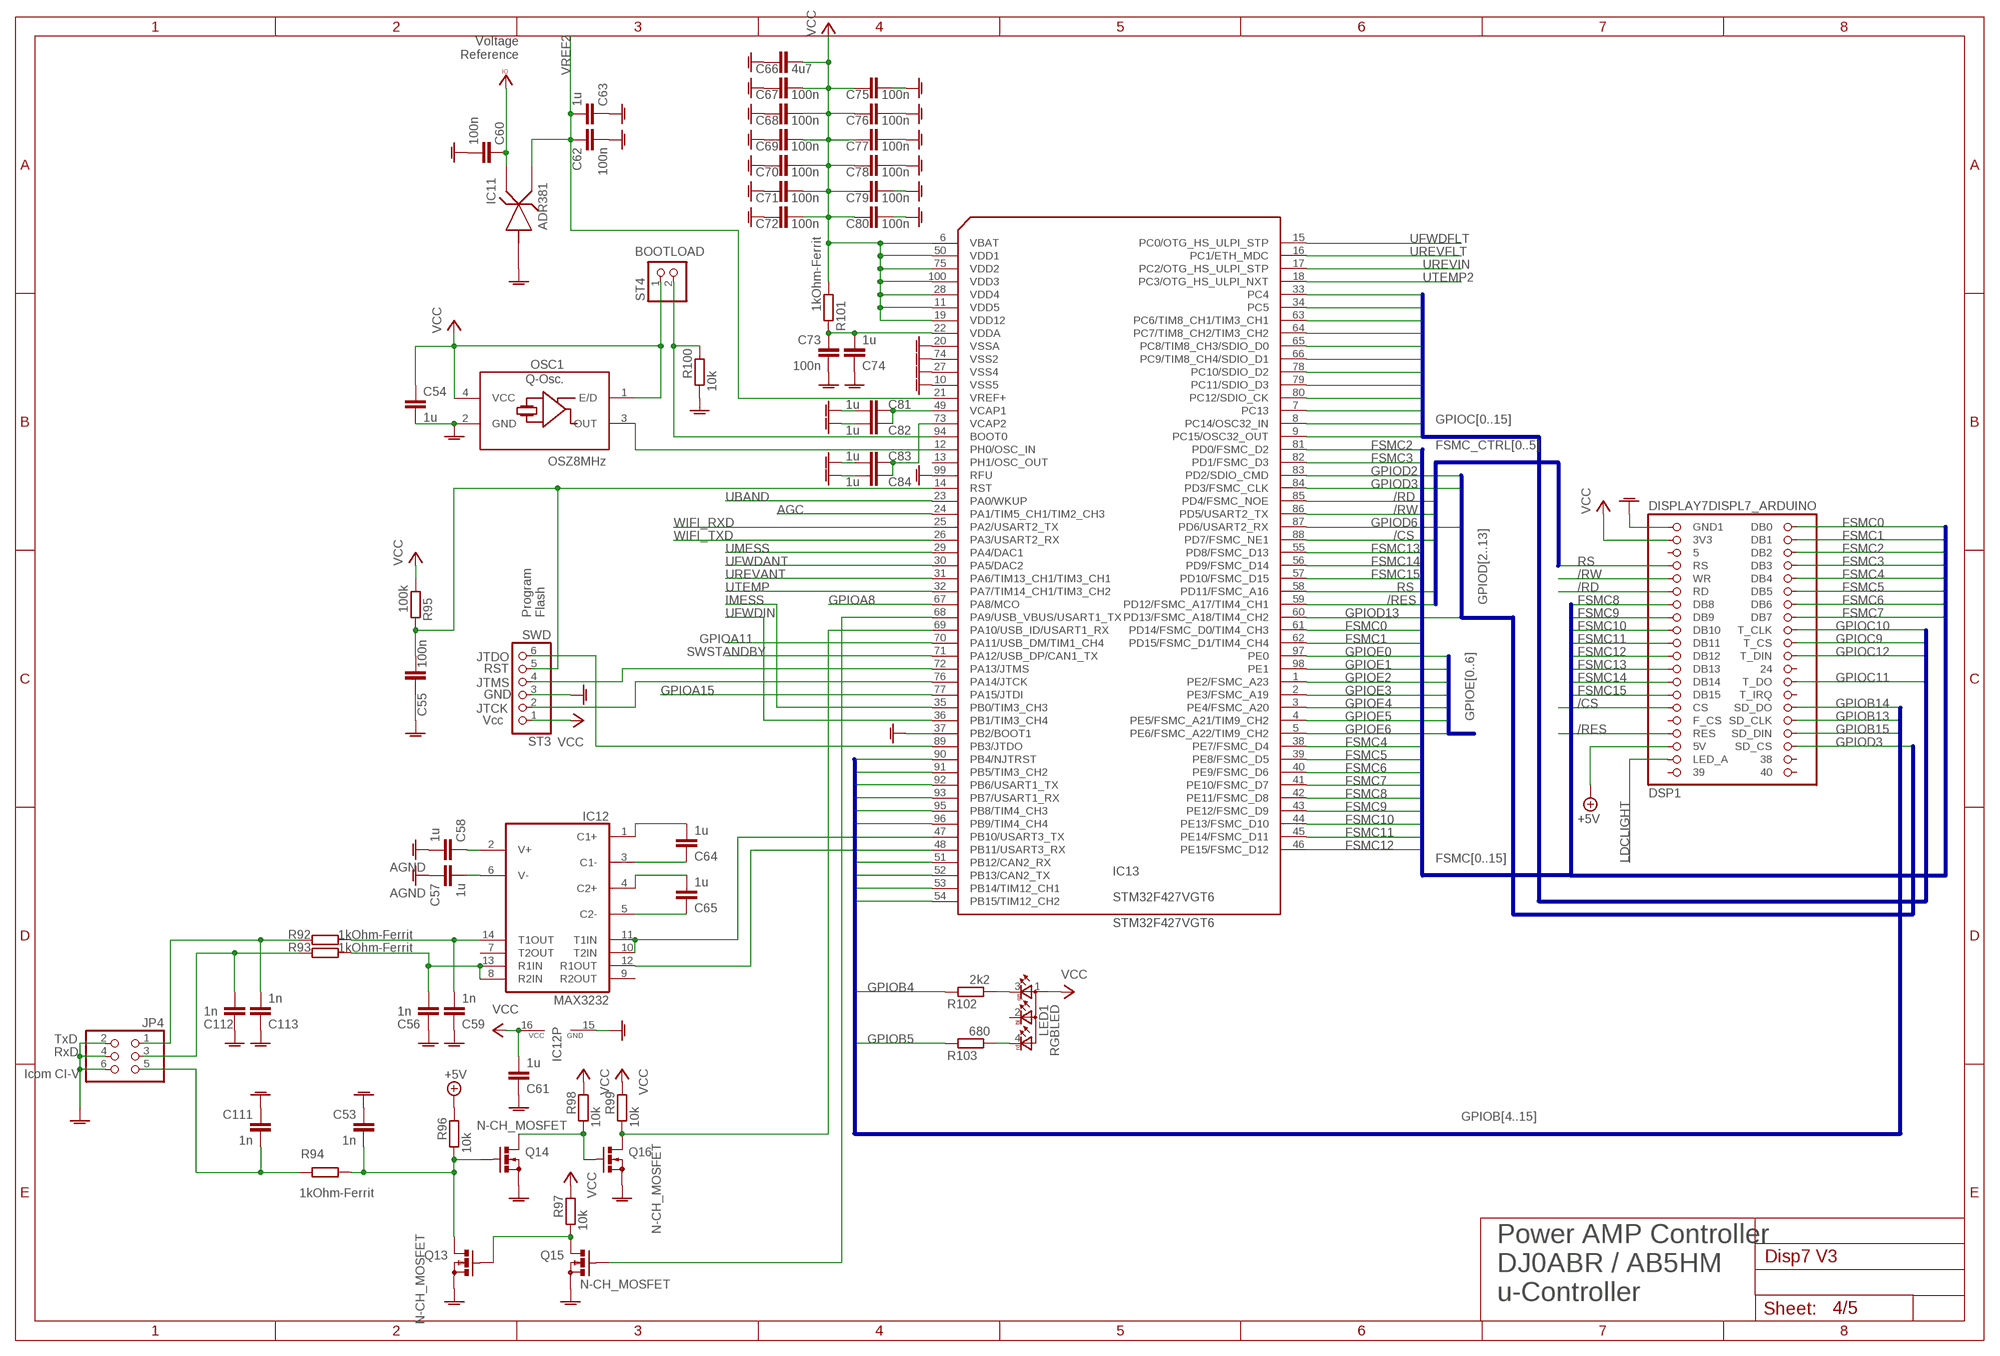
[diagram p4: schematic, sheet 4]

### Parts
C53  1n  C-EUC0805  [C0805]
C54  1u  C-EUC0805  [C0805]
C55  100n  C-EUC0805  [C0805]
C56  1n  C-EUC0805  [C0805]
C57  1u  C-EUC0805  [C0805]
C58  1u  C-EUC0805  [C0805]
C59  1n  C-EUC0805  [C0805]
C60  100n  C-EUC0805  [C0805]
C61  1u  C-EUC0805  [C0805]
C62  100n  C-EUC0805  [C0805]
C63  1u  C-EUC0805  [C0805]
C64  1u  C-EUC0805  [C0805]
C65  1u  C-EUC0805  [C0805]
C66  4u7  C-EUC0805  [C0805]
C67  100n  C-EUC0805  [C0805]
C68  100n  C-EUC0805  [C0805]
C69  100n  C-EUC0805  [C0805]
C70  100n  C-EUC0805  [C0805]
C71  100n  C-EUC0805  [C0805]
C72  100n  C-EUC0805  [C0805]
C73  100n  C-EUC0805  [C0805]
C74  1u  C-EUC0805  [C0805]
C75  100n  C-EUC0805  [C0805]
C76  100n  C-EUC0805  [C0805]
C77  100n  C-EUC0805  [C0805]
C78  100n  C-EUC0805  [C0805]
C79  100n  C-EUC0805  [C0805]
C80  100n  C-EUC0805  [C0805]
C81  1u  C-EUC0805  [C0805]
C82  1u  C-EUC0805  [C0805]
C83  1u  C-EUC0805  [C0805]
C84  1u  C-EUC0805  [C0805]
C111  1n  C-EUC0805  [C0805]
C112  1n  C-EUC0805  [C0805]
C113  1n  C-EUC0805  [C0805]
DSP1  DISPLAY7DISPL7_ARDUINO  [2X20]
IC11  ADR381  LT1004  [SOT23@1]
IC12  MAX3232  MAX3232CSE  [SO16]
IC13  STM32F427VGT6  STM32F205VG  [TQFP100]
JP4  PINHD-2X3/90  [2X03/90]
LED1  RGBLED  LED_RGB_WE  [PLCC4_WE_LED]
OSC1  OSZ8MHz  QOSC_AURELAURIS7050  [QOSC_AQO7015]
Q13  N-CH_MOSFET  BS170_SMD  [SOT23]
Q14  N-CH_MOSFET  BS170_SMD  [SOT23]
Q15  N-CH_MOSFET  BS170_SMD  [SOT23]
Q16  N-CH_MOSFET  BS170_SMD  [SOT23]
R92  1kOhm-Ferrit  R-EU_R0805  [R0805]
R93  1kOhm-Ferrit  R-EU_R0805  [R0805]
R94  1kOhm-Ferrit  R-EU_R0805  [R0805]
R95  100k  R-EU_R0805  [R0805]
R96  10k  R-EU_R0603  [R0603]
R97  10k  R-EU_R0805  [R0805]
R98  10k  R-EU_R0805  [R0805]
R99  10k  R-EU_R0805  [R0805]
R100  10k  R-EU_R0805  [R0805]
R101  1kOhm-Ferrit  R-EU_R0805  [R0805]
R102  2k2  R-EU_R0805  [R0805]
R103  680  R-EU_R0805  [R0805]
ST3  SWD  PINHEAD6X1P6  [PINHEAD6X1]
ST4  PINHEAD2X1SMALL  [PINHEAD1X2]

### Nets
+5V: DSP1.35(5V) R96.2 ; also sheet 1,3
/CS: DSP1.29(CS) IC13.88(PD7/FSMC_NE1)
/RD: DSP1.11(RD) IC13.85(PD4/FSMC_NOE)
/RES: DSP1.33(RES) IC13.59(PD12/FSMC_A17/TIM4_CH1)
/RW: DSP1.9(WR) IC13.86(PD5/USART2_TX)
AGC: IC13.24(PA1/TIM5_CH1/TIM2_CH3) ; also sheet 3
AGND [AGND]: C53.1 C54.2 C55.1 C56.1 C57.1 C58.2 C59.1 C60.2 C61.1 C62.2 C63.1 C66.1 C67.1 C68.1 C69.1 C70.1 C71.1 C72.1 C73.2 C74.1 C75.2 C76.2 C77.2 C78.2 C79.2 C80.2 C81.1 C82.1 C83.1 C84.1 C111.1 C112.1 C113.1 DSP1.1(GND1) IC11.3(A) IC12.15(GND) IC13.10(VSS5) IC13.20(VSSA) IC13.27(VSS4) IC13.37(PB2/BOOT1) IC13.74(VSS2) IC13.99(RFU) JP4.2 JP4.4 JP4.6 OSC1.2(GND) Q13.2(S) Q14.2(S) Q15.2(S) Q16.2(S) R100.1 ST3.3 ; supply symbol labelled  ; also sheet 1,2,3,5
FSMC0: DSP1.2(DB0) IC13.61(PD14/FSMC_D0/TIM4_CH3)
FSMC1: DSP1.4(DB1) IC13.62(PD15/FSMC_D1/TIM4_CH4)
FSMC2: DSP1.6(DB2) IC13.81(PD0/FSMC_D2)
FSMC3: DSP1.8(DB3) IC13.82(PD1/FSMC_D3)
FSMC4: DSP1.10(DB4) IC13.38(PE7/FSMC_D4)
FSMC5: DSP1.12(DB5) IC13.39(PE8/FSMC_D5)
FSMC6: DSP1.14(DB6) IC13.40(PE9/FSMC_D6)
FSMC7: DSP1.16(DB7) IC13.41(PE10/FSMC_D7)
FSMC8: DSP1.13(DB8) IC13.42(PE11/FSMC_D8)
FSMC9: DSP1.15(DB9) IC13.43(PE12/FSMC_D9)
FSMC10: DSP1.17(DB10) IC13.44(PE13/FSMC_D10)
FSMC11: DSP1.19(DB11) IC13.45(PE14/FSMC_D11)
FSMC12: DSP1.21(DB12) IC13.46(PE15/FSMC_D12)
FSMC13: DSP1.23(DB13) IC13.55(PD8/FSMC_D13)
FSMC14: DSP1.25(DB14) IC13.56(PD9/FSMC_D14)
FSMC15: DSP1.27(DB15) IC13.57(PD10/FSMC_D15)
GPIOA8: IC13.67(PA8/MCO)
GPIOA11: IC13.70(PA11/USB_DM/TIM1_CH4) ; also sheet 2
GPIOA15: IC13.77(PA15/JTDI)
GPIOB4: IC13.90(PB4/NJTRST) R102.2
GPIOB5: IC13.91(PB5/TIM3_CH2) R103.2
GPIOB6: IC13.92(PB6/USART1_TX) ; also sheet 2
GPIOB7: IC13.93(PB7/USART1_RX) ; also sheet 2
GPIOB8: IC13.95(PB8/TIM4_CH3) ; also sheet 2
GPIOB9: IC13.96(PB9/TIM4_CH4) ; also sheet 2
GPIOB12: IC13.51(PB12/CAN2_RX) ; also sheet 2
GPIOB13: DSP1.32(SD_CLK) IC13.52(PB13/CAN2_TX)
GPIOB14: DSP1.30(SD_DO) IC13.53(PB14/TIM12_CH1)
GPIOB15: DSP1.34(SD_DIN) IC13.54(PB15/TIM12_CH2)
GPIOC4: IC13.33(PC4) ; also sheet 2
GPIOC5: IC13.34(PC5) ; also sheet 2
GPIOC6: IC13.63(PC6/TIM8_CH1/TIM3_CH1)
GPIOC7: IC13.64(PC7/TIM8_CH2/TIM3_CH2)
GPIOC8: IC13.65(PC8/TIM8_CH3/SDIO_D0)
GPIOC9: DSP1.20(T_CS) IC13.66(PC9/TIM8_CH4/SDIO_D1)
GPIOC10: DSP1.18(T_CLK) IC13.78(PC10/SDIO_D2)
GPIOC11: DSP1.26(T_DO) IC13.79(PC11/SDIO_D3)
GPIOC12: DSP1.22(T_DIN) IC13.80(PC12/SDIO_CK)
GPIOC13: IC13.7(PC13) ; also sheet 2
GPIOC14: IC13.8(PC14/OSC32_IN) ; also sheet 2
GPIOC15: IC13.9(PC15/OSC32_OUT) ; also sheet 2
GPIOD2: IC13.83(PD2/SDIO_CMD) ; also sheet 2
GPIOD3: DSP1.36(SD_CS) IC13.84(PD3/FSMC_CLK)
GPIOD6: IC13.87(PD6/USART2_RX)
GPIOD13: IC13.60(PD13/FSMC_A18/TIM4_CH2) ; also sheet 2
GPIOE0: IC13.97(PE0) ; also sheet 2
GPIOE1: IC13.98(PE1) ; also sheet 2
GPIOE2: IC13.1(PE2/FSMC_A23) ; also sheet 2
GPIOE3: IC13.2(PE3/FSMC_A19) ; also sheet 2
GPIOE4: IC13.3(PE4/FSMC_A20) ; also sheet 2
GPIOE5: IC13.4(PE5/FSMC_A21/TIM9_CH2)
GPIOE6: IC13.5(PE6/FSMC_A22/TIM9_CH2) ; also sheet 2
IMESS: IC13.35(PB0/TIM3_CH3) ; also sheet 3
LDCLIGHT: DSP1.37(LED_A) ; also sheet 2
N$9: LED1.3(CRED) R102.1
N$13: C64.1 IC12.3(C1-)
N$15: C64.2 IC12.1(C1+)
N$28: C65.2 IC12.4(C2+)
N$30: C65.1 IC12.5(C2-)
N$31: C58.1 IC12.2(V+)
N$32: C57.2 IC12.6(V-)
N$34: IC12.10(T2IN) IC12.11(T1IN) IC13.47(PB10/USART3_TX)
N$35: C59.2 IC12.14(T1OUT) R92.2
N$36: C53.2 Q13.3(D) Q14.1(G) R94.2 R96.1
N$37: IC12.12(R1OUT) IC13.48(PB11/USART3_RX)
N$39: Q14.3(D) Q16.1(G) R98.1
N$40: IC13.69(PA10/USB_ID/USART1_RX) Q16.3(D) R99.1
N$41: C56.2 IC12.8(R2IN) IC12.13(R1IN) R93.2
N$42: IC13.68(PA9/USB_VBUS/USART1_TX) Q15.1(G)
N$43: Q13.1(G) Q15.3(D) R97.1
N$48: LED1.4(CGREEN) R103.1
N$77: C113.2 JP4.1 R92.1
N$84: C112.2 JP4.3 R93.1
N$87: C111.2 JP4.5 R94.1
N$117: C83.2 C84.2 IC13.73(VCAP2)
N$153: IC13.12(PH0/OSC_IN) OSC1.3(OUT)
N$154: C81.2 C82.2 IC13.49(VCAP1)
N$156: C73.1 C74.2 IC13.22(VDDA) R101.2
N$157: C55.2 IC13.14(RST) R95.2 ST3.5
N$158: IC13.94(BOOT0) R100.2 ST4.2
N$159: IC13.76(PA14/JTCK) ST3.2
N$160: IC13.72(PA13/JTMS) ST3.4
N$161: IC13.89(PB3/JTDO) ST3.6
RS: DSP1.7(RS) IC13.58(PD11/FSMC_A16)
SWSTANDBY: IC13.71(PA12/USB_DP/CAN1_TX)
UBAND: IC13.23(PA0/WKUP) ; also sheet 3
UFWDANT: IC13.30(PA5/DAC2) ; also sheet 3
UFWDFLT: IC13.15(PC0/OTG_HS_ULPI_STP) ; also sheet 3
UFWDIN: IC13.36(PB1/TIM3_CH4) ; also sheet 3
UMESS: IC13.29(PA4/DAC1) ; also sheet 3
UREVANT: IC13.31(PA6/TIM13_CH1/TIM3_CH1) ; also sheet 3
UREVFLT: IC13.16(PC1/ETH_MDC) ; also sheet 3
UREVIN: IC13.17(PC2/OTG_HS_ULPI_STP) ; also sheet 3
UTEMP: IC13.32(PA7/TIM14_CH1/TIM3_CH2) ; also sheet 3
UTEMP2: IC13.18(PC3/OTG_HS_ULPI_NXT) ; also sheet 3
VCC [Supply]: C54.1 C61.2 C66.2 C67.2 C68.2 C69.2 C70.2 C71.2 C72.2 C75.1 C76.1 C77.1 C78.1 C79.1 C80.1 DSP1.3(3V3) IC12.16(VCC) IC13.6(VBAT) IC13.11(VDD5) IC13.19(VDD12) IC13.28(VDD4) IC13.50(VDD1) IC13.75(VDD2) IC13.100(VDD3) LED1.1(A2) OSC1.1(E/D) OSC1.4(VCC) R95.1 R97.2 R98.2 R99.2 R101.1 ST3.1 ST4.1 ; also sheet 1,2,5
VCCIO [Supply]: C60.1 IC11.1(K2) ; supply symbol labelled  ; also sheet 1,3
VREF2: C62.1 C63.2 IC11.2(K1) IC13.21(VREF+) ; also sheet 3
WIFI_RXD: IC13.25(PA2/USART2_TX) ; also sheet 5
WIFI_TXD: IC13.26(PA3/USART2_RX) ; also sheet 5
Unconnected: DSP1.5 DSP1.24 DSP1.28(T_IRQ) DSP1.31(F_CS) DSP1.38 DSP1.39 DSP1.40 IC12.7(T2OUT) IC12.9(R2OUT) IC13.13(PH1/OSC_OUT) LED1.2(CBLUE)

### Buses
FSMC[0..15]
FSMC_CTRL[0..5]
GPIOC[0..15]
GPIOE[0..6]
GPIOD[2..13]
GPIOB[4..15]

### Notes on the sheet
- Voltage
  Reference
- BOOTLOAD
- Program
  Flash
- JTDO
- RST
- JTMS
- GND
- JTCK
- Vcc
- STM32F427VGT6
- TxD
- RxD
- Icom CI-V
- Power AMP Controller
  DJ0ABR / AB5HM
  u-Controller

## Sheet 5 of 5: WLAN IF
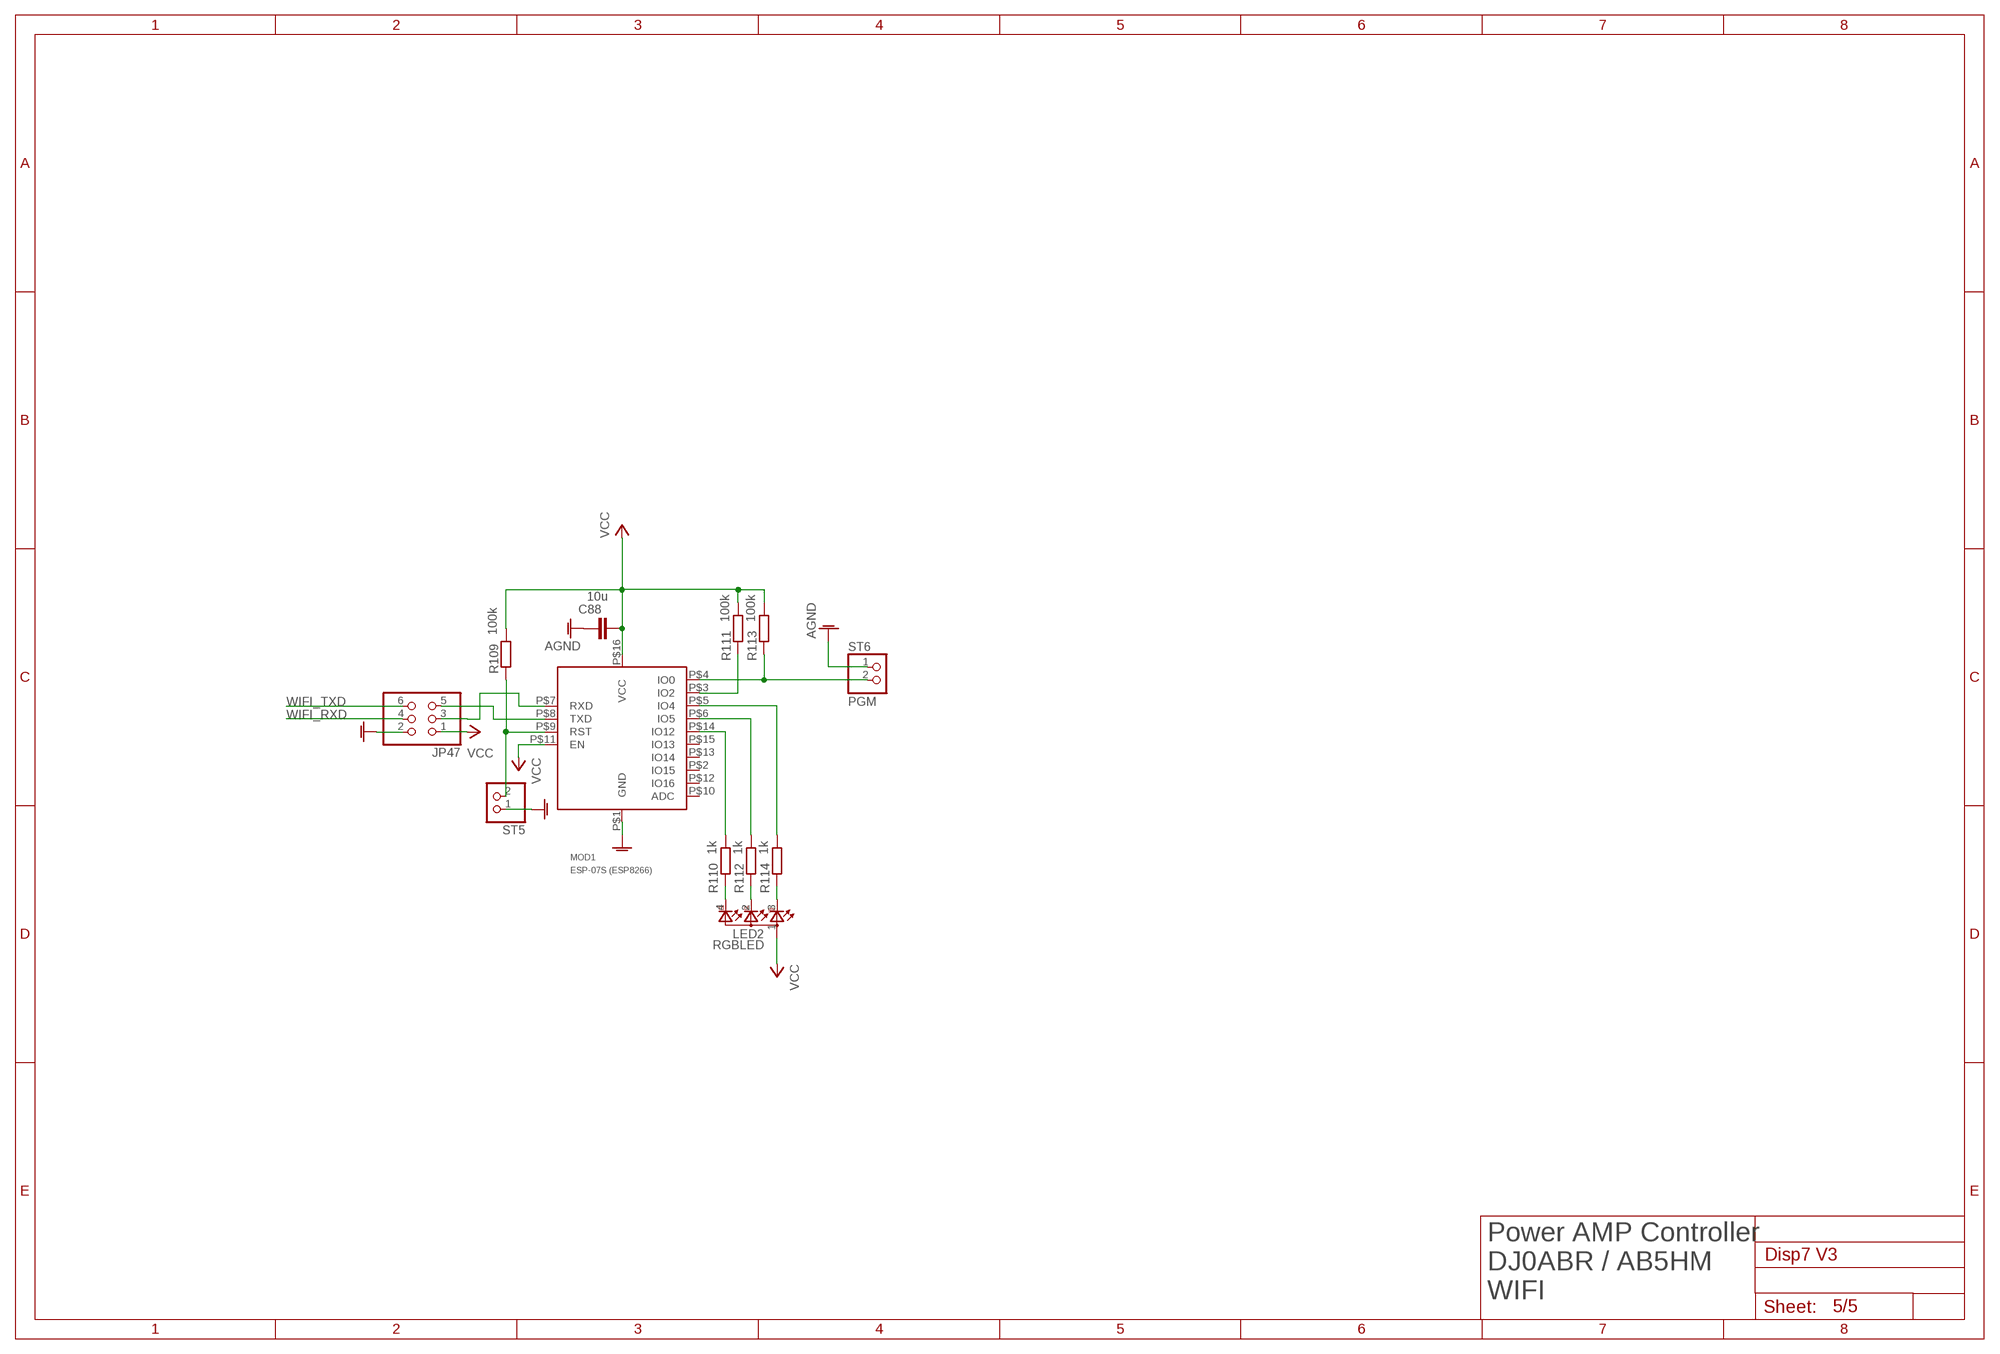
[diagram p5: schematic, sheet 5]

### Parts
C88  10u  C-EUC0805  [C0805]
JP47  PINHD-2X3  [2X03]
LED2  RGBLED  LED_RGB_WE  [PLCC4_WE_LED]
MOD1  ESP-07S (ESP8266)  ESP8266-1212  [ESP8266-12]
R109  100k  R-EU_R0805  [R0805]
R110  1k  R-EU_R0805  [R0805]
R111  100k  R-EU_R0805  [R0805]
R112  1k  R-EU_R0805  [R0805]
R113  100k  R-EU_R0805  [R0805]
R114  1k  R-EU_R0805  [R0805]
ST5  PINHEAD2X1BIG  [PINHEAD1X2BIG]
ST6  PGM  PINHEAD2X1SMALL  [PINHEAD1X2]

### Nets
AGND [AGND]: C88.1 JP47.2 MOD1.P$1(GND) ST5.1 ST6.1 ; supply symbol labelled  ; also sheet 1,2,3,4
N$16: MOD1.P$4(IO0) R113.1 ST6.2
N$17: LED2.3(CRED) R114.1
N$18: LED2.2(CBLUE) R112.1
N$20: LED2.4(CGREEN) R110.1
N$22: MOD1.P$14(IO12) R110.2
N$23: MOD1.P$6(IO5) R112.2
N$24: MOD1.P$9(RST) R109.1 ST5.2
N$25: MOD1.P$3(IO2) R111.1
N$26: MOD1.P$5(IO4) R114.2
N$101: JP47.3 MOD1.P$7(RXD)
N$102: JP47.5 MOD1.P$8(TXD)
VCC [Supply]: C88.2 JP47.1 LED2.1(A2) MOD1.P$11(EN) MOD1.P$16(VCC) R109.2 R111.2 R113.2 ; also sheet 1,2,4
WIFI_RXD: JP47.4 ; also sheet 4
WIFI_TXD: JP47.6 ; also sheet 4
Unconnected: MOD1.P$2(IO15) MOD1.P$10(ADC) MOD1.P$12(IO16) MOD1.P$13(IO14) MOD1.P$15(IO13)

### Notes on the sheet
- Power AMP Controller
  DJ0ABR / AB5HM
  WIFI

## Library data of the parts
C1 = rcl:CPOL-EU: POLARIZED CAPACITOR, European symbol
C2-C123 = rcl:C-EU: CAPACITOR, European symbol
D1 D9-D13 D18 = km:DIODE_GROSS
D2-D8 D14-D17 D19 = diode:DIODE-: DIODE
DSP1 = km:DISPLAY7
FID1 FID2 = km:FIDUCIAL
IC1 = v-reg:LP2950?*: Source: http://cache.national.com/ds/LP/LP2950.pdf
IC2 = km:78XX
IC3 = km:UREG5
IC4 = burr-brown:INA168: High-Side Measurement Current Shunt Monitor; MF: TEXAS INSTRUMENTS; MPN: INA168NA/250; OC_FARNELL: 4375737; OC_NEWARK: 35C1744
IC5-IC9 = linear:LM358: OP AMP also LM158; LM258; LM2904 Source: http://cache.national.com/ds/LM/LM158.pdf
IC10 = linear:TL081: OP AMP
IC11 = km:LT1004
IC12 = maxim:MAX3232*: True RS-232 Transceivers 3.0V to 5.5V, Low-Power up to 1Mbps, Using Four 0.1µF External Capacitors Source: http://pdfserv.maxim-ic.com/en/ds/MAX3222-MAX3241.pdf; MPN: MAX3232CSE; OC_FARNELL: 9725490; OC_NEWARK: 90C2890
IC13 = STM32F205VG:STM32F205VG
JP4 JP47 = pinhead:PINHD-2X3: PIN HEADER
JP5 = pinhead:PINHD-2X8: PIN HEADER
JP6 = pinhead:PINHD-2X10: PIN HEADER
JP7 = pinhead:PINHD-2X4: PIN HEADER
JP8 = pinhead:PINHD-2X6: PIN HEADER
L1 = WE-PD3:WE-PD3: SMD-Shielded Power Inductor WE-PD3; MPN: 74451147; OC_FARNELL: 1636065; OC_NEWARK: 08P2637; PACKAGE: Type S; SUPPLIER: Würth Elektronik eiSos GmbH
LED1 LED2 = km:LED_RGB_WE
MOD1 = km:ESP8266-12
OSC1 = km:QOSC_AUREL
Q1 = transistor-small-signal:BSS84: P-CHANNEL MOS FET
Q2-Q4 Q10 Q13-Q16 = km:BS170_: N-CHANNEL MOS FET
Q5-Q9 Q11 = transistor-power:IRLR120N
R1-R56 R58 R59 R62-R89 R91-R103 R109-R115 = rcl:R-EU_: RESISTOR, European symbol
R90 = km:MINIPOTI-S
ST3 = km:PINHEAD6X1
ST4-ST6 = km:PINHEAD2X1
U1 = km:TC7662AEPA: CONVERTER, DC-DC, HI VOLT
X1 = con-phoenix-508:MSTBV4: PHOENIX; MPN: MSTBV 2,5/4-GF-5.08; OC_FARNELL: 1792794; OC_NEWARK: 69R9847
X2 = con-phoenix-508:MSTBV2: PHOENIX; MPN: MSTBV 2,5/2-GF-5.08; OC_FARNELL: 1792792; OC_NEWARK: 69R9845

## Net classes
0 default: drill 0.3 mm
1 Supply: width 0.203 mm, drill 0.3 mm, clearance 0.178 mm
2 v12: drill 0.3 mm
3 v533: drill 0.3 mm
4 AGND: width 0.152 mm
